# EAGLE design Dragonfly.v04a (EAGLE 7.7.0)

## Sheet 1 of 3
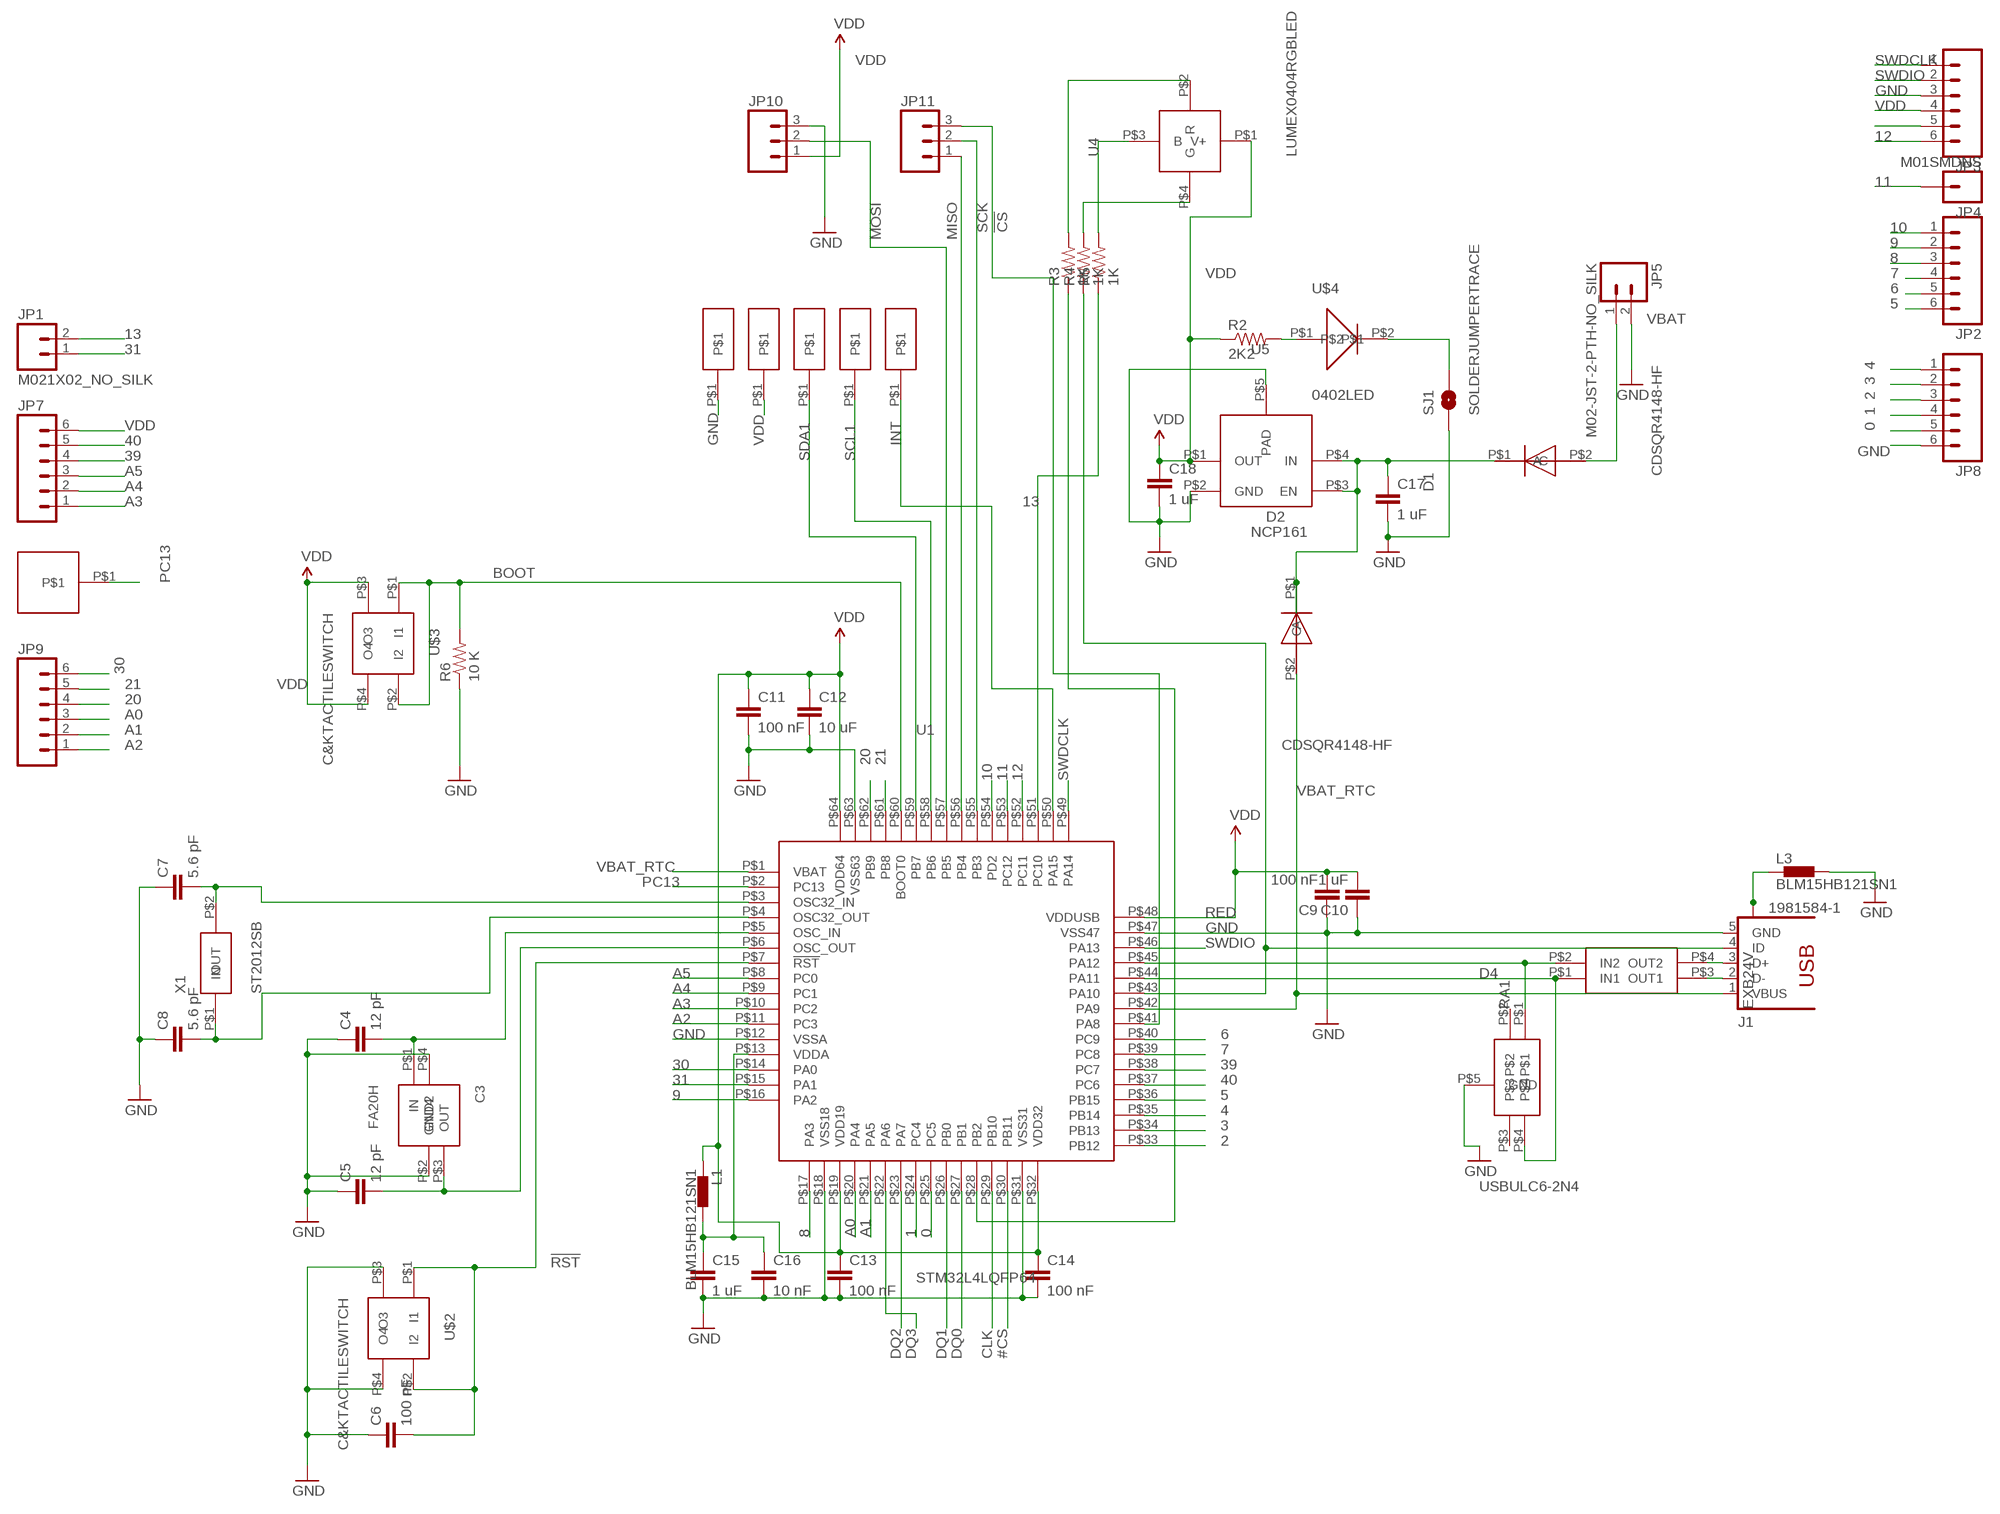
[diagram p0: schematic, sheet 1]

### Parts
C3  FA20H  [FA-20H]
C4  12 pF  0402CAP.KW  [0402-CAP]
C5  12 pF  0402CAP.KW  [0402-CAP]
C6  100 nF  0402CAP.KW  [0402-CAP]
C7  5.6 pF  0402CAP.KW  [0402-CAP]
C8  5.6 pF  0402CAP.KW  [0402-CAP]
C9  100 nF  0402CAP.KW  [0402-CAP]
C10  1 uF  0402CAP.KW  [0402-CAP]
C11  100 nF  0402CAP.KW  [0402-CAP]
C12  10 uF  0402CAP.KW  [0402-CAP]
C13  100 nF  0402CAP.KW  [0402-CAP]
C14  100 nF  0402CAP.KW  [0402-CAP]
C15  1 uF  0402CAP.KW  [0402-CAP]
C16  10 nF  0402CAP.KW  [0402-CAP]
C17  1 uF  0402CAP.KW  [0402-CAP]
C18  1 uF  0402CAP.KW  [0402-CAP]
D1  CDSQR4148-HF  [CDSQR4148-HF]
D2  CDSQR4148-HF  [CDSQR4148-HF]
D4  USBULC6-2N4  [USBULC6-2N4]
J1  1981584-1  [1981584-1]
JP1  M021X02_NO_SILK  [1X02_NO_SILK]
JP2  M06NO_SILK  [1X06_NO_SILK]
JP3  M06NO_SILK  [1X06_NO_SILK]
JP4  M01SMDNS  [1X01NS]
JP5  M02-JST-2-PTH-NO_SILK  [JST-2-PTH-NS]
JP7  M06NO_SILK  [1X06_NO_SILK]
JP8  M06NO_SILK  [1X06_NO_SILK]
JP9  M06NO_SILK  [1X06_NO_SILK]
JP10  M031X03_NO_SILK  [1X03_NO_SILK]
JP11  M031X03_NO_SILK  [1X03_NO_SILK]
L1  BLM15HB121SN1  [0402]
L3  BLM15HB121SN1  [0402]
R2  2K2  0402RES.KW  [0402-RES]
R3  1K  0402RES.KW  [0402-RES]
R4  1K  0402RES.KW  [0402-RES]
R5  1K  0402RES.KW  [0402-RES]
R6  10 K  0402RES.KW  [0402-RES]
RA1  EXB24V  [EXB24V]
SJ1  SOLDERJUMPERTRACE  [SJ_2S-TRACE]
U1  STM32L4LQFP64  [STM32L4LQFP64]
U4  LUMEX0404RGBLED  [LX0404]
U5  NCP161  [NCP161]
U$1  HN01  [HN01]
U$2  C&KTACTILESWITCH  [C&KTACTILESWITCH]
U$3  C&KTACTILESWITCH  [C&KTACTILESWITCH]
U$4  0402LED  [0402LED]
U$5  SMDPAD  [SMDPAD]
U$6  SMDPAD  [SMDPAD]
U$7  SMDPAD  [SMDPAD]
U$8  SMDPAD  [SMDPAD]
U$9  SMDPAD  [SMDPAD]
X1  ST2012SB  [ST2012SB]

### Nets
0: JP8.5 U1.P$25(PC5)
1: JP8.4 U1.P$24(PC4)
2: JP8.3 U1.P$33(PB12)
3: JP8.2 U1.P$34(PB13)
4: JP8.1 U1.P$35(PB14)
5: JP2.6 U1.P$36(PB15)
6: JP2.5 U1.P$40(PC9)
7: JP2.4 U1.P$39(PC8)
8: JP2.3 U1.P$17(PA3)
9: JP2.2 U1.P$16(PA2)
10: JP2.1 U1.P$54(PD2)
11: JP4.1 U1.P$53(PC12)
12: JP3.6 U1.P$52(PC11)
13: JP1.2 R5.1 U1.P$51(PC10)
20: JP9.4 U1.P$62(PB9)
21: JP9.5 U1.P$61(PB8)
30: JP9.6 U1.P$14(PA0)
31: JP1.1 U1.P$15(PA1)
39: JP7.4 U1.P$38(PC7)
40: JP7.5 U1.P$37(PC6)
!CS: JP11.3 U1.P$41(PA8)
!RST: C6.2 U1.P$7(!RST) U$2.P$1(I1) U$2.P$2(I2)
#CS: U1.P$30(PB11) ; also sheet 3
A0: JP9.3 U1.P$20(PA4)
A1: JP9.2 U1.P$21(PA5)
A2: JP9.1 U1.P$11(PC3)
A3: JP7.1 U1.P$10(PC2)
A4: JP7.2 U1.P$9(PC1)
A5: JP7.3 U1.P$8(PC0)
BOOT: R6.2 U1.P$60(BOOT0) U$3.P$1(I1) U$3.P$2(I2)
CLK: U1.P$29(PB10) ; also sheet 3
DQ0: U1.P$27(PB1) ; also sheet 3
DQ1: U1.P$26(PB0) ; also sheet 3
DQ2: U1.P$23(PA7) ; also sheet 3
DQ3: U1.P$22(PA6) ; also sheet 3
GND: C3.P$2(GND2) C3.P$4(GND4) C4.1 C5.1 C6.1 C7.1 C8.1 C9.1 C10.1 C11.2 C12.2 C13.2 C14.2 C15.2 C16.2 C17.2 C18.2 D4.P$5(GND) J1.5(GND) JP3.3 JP5.2 JP8.6 JP10.3 L3.2 R6.1 SJ1.1 U1.P$12(VSSA) U1.P$18(VSS18) U1.P$31(VSS31) U1.P$47(VSS47) U1.P$63(VSS63) U5.P$2(GND) U5.P$5(PAD) U$2.P$3(O3) U$2.P$4(O4) U$7.P$1 ; also sheet 3
INT: U1.P$50(PA15) U$9.P$1
MISO: JP11.1 U1.P$56(PB4)
MOSI: JP10.2 U1.P$57(PB5)
N$1: C7.2 U1.P$3(OSC32_IN) X1.P$2(OUT)
N$2: C8.2 U1.P$4(OSC32_OUT) X1.P$1(IN)
N$3: C3.P$1(IN) C4.2 U1.P$5(OSC_IN)
N$4: C3.P$3(OUT) C5.2 U1.P$6(OSC_OUT)
N$9: C15.1 C16.1 L1.2 U1.P$13(VDDA)
N$11: R3.2 U4.P$2(R)
N$13: SJ1.2 U$4.P$2
N$31: J1.3(D+) RA1.P$4(OUT2)
N$32: J1.4(ID) R4.1 U1.P$43(PA10)
N$33: J1.2(D-) RA1.P$3(OUT1)
N$38: D4.P$1 RA1.P$2(IN2) U1.P$45(PA12)
N$39: D4.P$4 RA1.P$1(IN1) U1.P$44(PA11)
N$42: R2.2 U$4.P$1
N$49: D2.P$2(A) J1.1(VBUS) U1.P$42(PA9)
N$56: R4.2 U4.P$4(G)
N$59: R5.2 U4.P$3(B)
N$60: C17.1 D1.P$1(C) D2.P$1(C) U5.P$3(EN) U5.P$4(IN)
PC13: U1.P$2(PC13) U$1.P$1
RED: R3.1 U1.P$28(PB2)
SCK: JP11.2 U1.P$55(PB3)
SCL1: U1.P$58(PB6) U$6.P$1
SDA1: U1.P$59(PB7) U$5.P$1
SWDCLK: JP3.1 U1.P$49(PA14)
SWDIO: JP3.2 U1.P$46(PA13)
USB_SHIELD: J1.S1 J1.S2 J1.S3 J1.S4 L3.1
VBAT: D1.P$2(A) JP5.1
VBAT_RTC: JP3.5 U1.P$1(VBAT)
VDD: C9.2 C10.2 C11.1 C12.1 C13.1 C14.1 C18.1 JP3.4 JP7.6 JP10.1 L1.1 R2.1 U1.P$19(VDD19) U1.P$32(VDD32) U1.P$48(VDDUSB) U1.P$64(VDD64) U4.P$1(V+) U5.P$1(OUT) U$3.P$3(O3) U$3.P$4(O4) U$8.P$1 ; also sheet 3
Unconnected: D4.P$2 D4.P$3

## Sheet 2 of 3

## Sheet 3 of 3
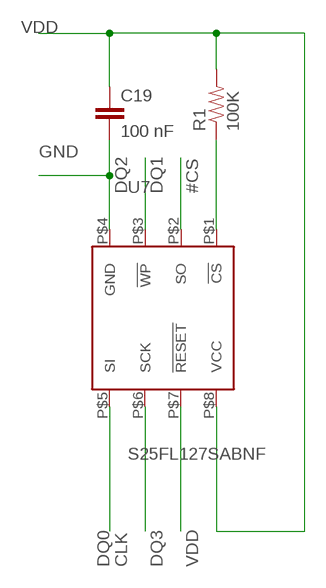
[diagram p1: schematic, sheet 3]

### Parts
C19  100 nF  0402CAP.KW  [0402-CAP]
R1  100K  0402RES.KW  [0402-RES]
U7  S25FL127SABNF  [WSON-8]

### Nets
#CS: R1.1 U7.P$1(!CS) ; also sheet 1
CLK: U7.P$6(SCK) ; also sheet 1
DQ0: U7.P$5(SI) ; also sheet 1
DQ1: U7.P$2(SO) ; also sheet 1
DQ2: U7.P$3(!WP) ; also sheet 1
DQ3: U7.P$7(!RESET) ; also sheet 1
GND: C19.2 U7.P$4(GND) ; also sheet 1
VDD: C19.1 R1.2 U7.P$8(VCC) ; also sheet 1

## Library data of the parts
C3 = Kris:FA20H: Seiko Epson 2.5 mm x 2.0 mm FA-20H 16 MHz crystal
C4-C19 = SparkFun-Capacitors:0402CAP.KW
D1 D2 = Kris:CDSQR4148-HF: ComChip's CDSQR4148-HF high speed 150 mA Io diode
D4 = Kris:USBULC6-2N4: ST TVS diode ESD Protection USBULC6-2N4
J1 = con-usb:1981584-1: Receptacle, micro-USB, type A/B Tyco Electronics; MF: Hirose; MPN: ZX62-AB-5PA(11)
JP1 JP5 = SparkFun-Connectors:M02: Standard 2-pin 0.1" header. Use with
JP2 JP3 JP7-JP9 = SparkFun-Connectors:M06: Header 6 Standard 6-pin 0.1" header. Use with straight break away headers (SKU : PRT-00116), right angle break away headers (PRT-00553), swiss pins (PRT-00743), machine pins (PRT-00117), and female headers (PRT-00115). Molex polarized connector foot print use with SKU : PRT-08094 with associated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
JP4 = SparkFun-Connectors:M01: Header 1
JP10 JP11 = SparkFun-Connectors:M03: Header 3 Standard 3-pin 0.1" header. Use with straight break away headers (SKU : PRT-00116), right angle break away headers (PRT-00553), swiss pins (PRT-00743), machine pins (PRT-00117), and female headers (PRT-00115). Molex polarized connector foot print use with SKU : PRT-08232 with associated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
L1 L3 = inductors:BLM15H: EMIFIL (R) Chip Ferrite Bead for GHz Noise
R1-R6 = SparkFun-Resistors:0402RES.KW
RA1 = Kris:EXB24V: Panasonic EXB24 22 Ohm series resistor pair
SJ1 = SparkFun-Passives:SOLDERJUMPER: Solder Jumper
U1 = Kris:STM32L4LQFP64: LQFP64 Package for ST's STM32L476 32-bit low-power microcontroller
U4 = Kris:LUMEX0404RGBLED: Lumex 0404 rgb leds
U5 = Kris:NCP161: NCP161 3V3 LDO voltage regulator
U7 = Kris:S25FL127SABNF: S225FL127SABNF1101 128 Mbit Spansion flash in WSON-8 package
U$1 = PWSONN6:HN01
U$2 U$3 = Kris:C&KTACTILESWITCH: C&K Tactile Switch 611-PTS810SJS250SMTR
U$4 = Kris:0402LED: 0402led
U$5-U$9 = Kris:SMDPAD: smd test pad
X1 = Kris:ST2012SB: Kyocera 2.0 x 1.2 mm 32.768 20kHz ppm 4 pf crystal

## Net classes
1 USB: width 0.254 mm, drill 0.33 mm, clearance 0.159 mm
2 Top GND Pour: clearance 0.762 mm to class 1

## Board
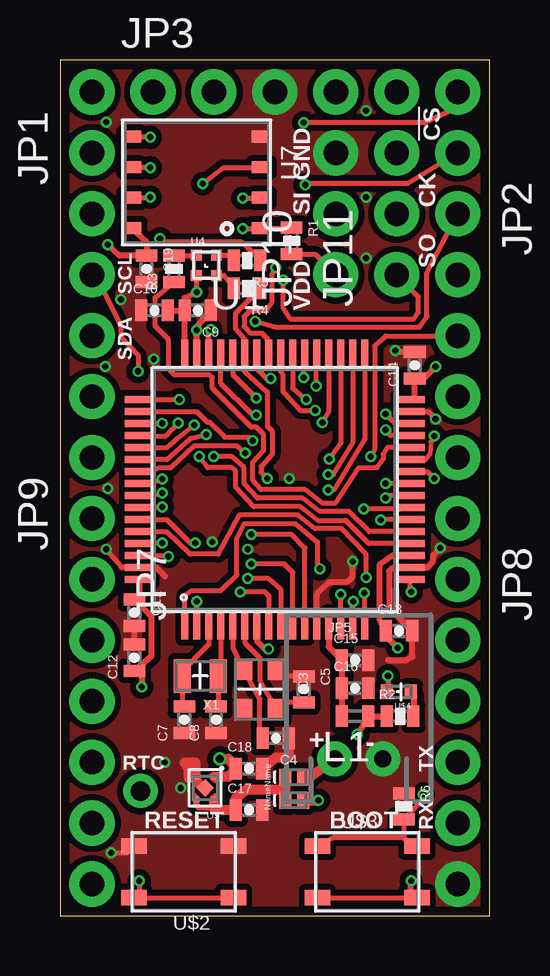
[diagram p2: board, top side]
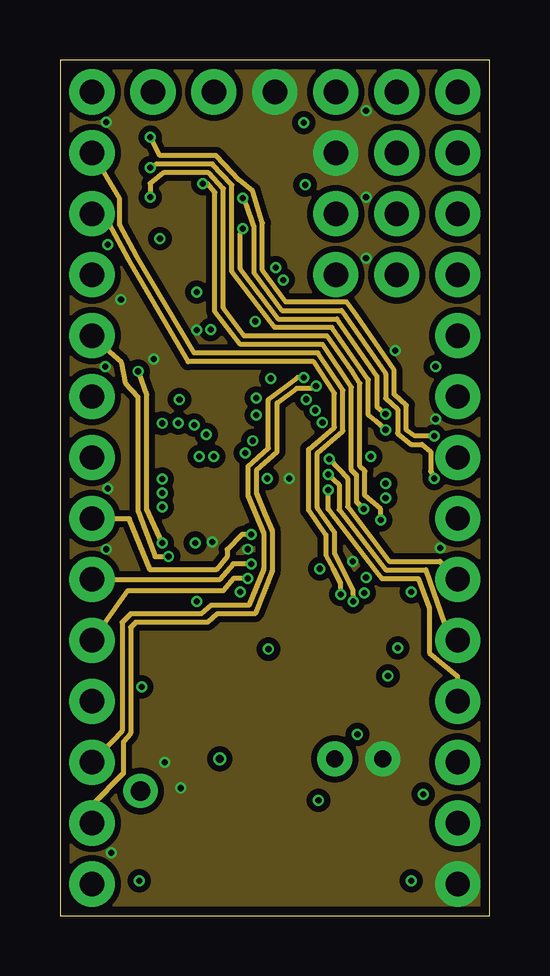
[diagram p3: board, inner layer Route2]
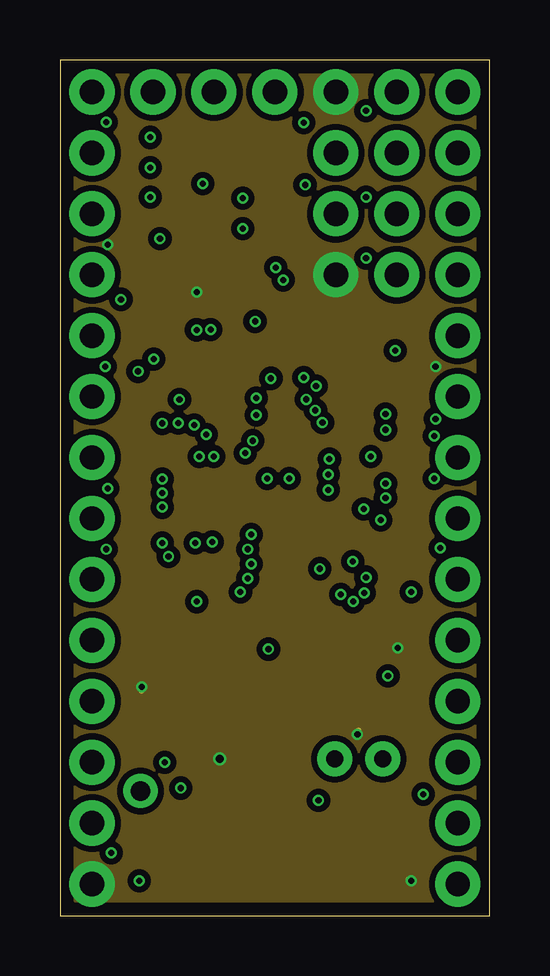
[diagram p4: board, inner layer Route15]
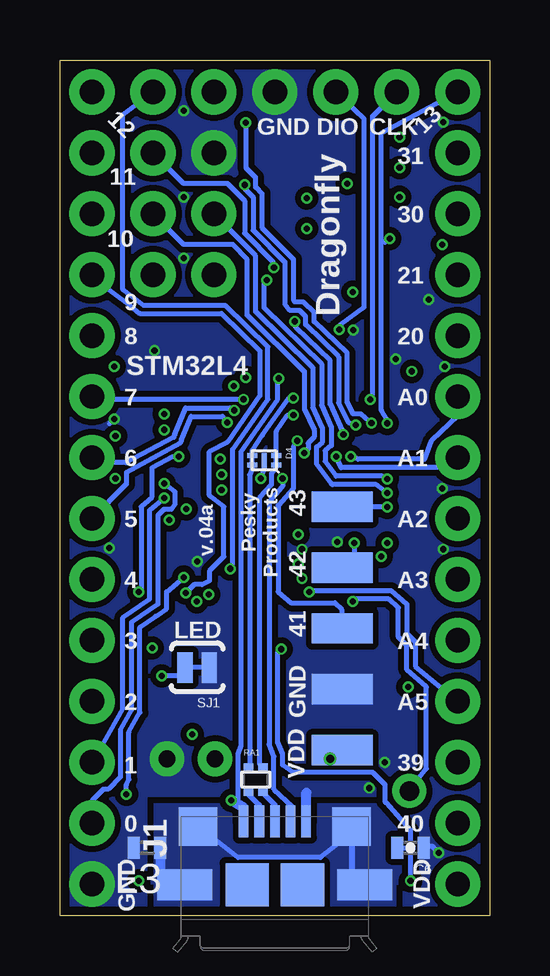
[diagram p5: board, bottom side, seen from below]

Size 17.91 x 35.69 mm. Coordinates in mm from the lower left corner, seen from the top.
Outline: 0,0 17.91,0 17.91,35.69 0,35.69 0,0
Copper layers (1*2*15*16): Top 0.035559375mm / dielectric 0.17018125mm / Route2 0.01778125mm / dielectric 47mil / Route15 0.01778125mm / dielectric 0.17018125mm / Bottom 0.035559375mm
Design rules "OSHPark-4layer *": minimum track width 5mil, minimum drill 10mil, track to track 5mil, track to pad 5mil, pad to pad 5mil, via to via 5mil, smd to smd 5mil, copper to edge 15mil, drill to drill 6mil, minimum pad ring 4mil, minimum via ring 4mil, stop-mask expansion 4mil, vias tented up to drill 20mil, thermal gap 10mil

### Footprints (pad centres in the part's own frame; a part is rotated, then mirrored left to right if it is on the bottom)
FA-20H = smd 0.9 x 0.75: P$1 -0.85,-0.7; P$2 0.85,-0.7; P$3 0.85,0.7; P$4 -0.85,0.7
0402-CAP = smd 0.5 x 0.9: 1 -0.55,0; 2 0.55,0
CDSQR4148-HF = smd 0.7 x 0.5: P$1 0,0.375; P$2 0,-0.375
USBULC6-2N4 = smd 0.2 x 0.4: P$1 0.2,0.5; P$2 -0.2,0.5; P$3 -0.2,-0.5; P$4 0.2,-0.5 | smd 0.6 x 0.2: P$5 0,0
1981584-1 = smd 0.4 x 1.35: 1 -1.3,4.1; 2 -0.65,4.1; 3 0,4.1; 4 0.65,4.1; 5 1.3,4.1 | smd 1.8 x 1.8: M1 -1.15,1.45; M2 1.15,1.45 | smd 2.3 x 1.3: S1 -3.75,1.45; S2 3.75,1.45 | smd 1.6 x 1.6: S3 -3.2,3.885; S4 3.2,3.885
1X02_NO_SILK = drill 1.016 pad 1.88: 1 0,0; 2 2.54,0
1X06_NO_SILK = drill 1.016 pad 1.88: 1 0,0; 2 2.54,0; 3 5.08,0; 4 7.62,0; 5 10.16,0; 6 12.7,0
1X01NS = drill 1.016 pad 1.88: 1 0,0
JST-2-PTH-NS = drill 0.7 pad 1.448: 1 -1,0; 2 1,0
1X03_NO_SILK = drill 1.016 pad 1.88: 1 0,0; 2 2.54,0; 3 5.08,0
0402 = smd 0.5 x 0.9: 1 -0.55,0; 2 0.55,0
0402-RES = smd 0.5 x 0.9: 1 -0.55,0; 2 0.55,0
EXB24V = smd 0.4 x 0.36: P$1 -0.3,0.5; P$2 0.3,0.5; P$3 -0.3,-0.5; P$4 0.3,-0.5
SJ_2S-TRACE = smd 0.635 x 1.27: 1 -0.508,0; 2 0.508,0
STM32L4LQFP64 = smd 0.3 x 1.2: P$1 -3.75,-5.65; P$2 -3.25,-5.65; P$3 -2.75,-5.65; P$4 -2.25,-5.65; P$5 -1.75,-5.65; P$6 -1.25,-5.65; P$7 -0.75,-5.65; P$8 -0.25,-5.65; P$9 0.25,-5.65; P$10 0.75,-5.65; P$11 1.25,-5.65; P$12 1.75,-5.65; P$13 2.25,-5.65; P$14 2.75,-5.65; P$15 3.25,-5.65; P$16 3.75,-5.65; P$33 3.75,5.65; P$34 3.25,5.65; P$35 2.75,5.65; P$36 2.25,5.65; P$37 1.75,5.65; P$38 1.25,5.65; P$39 0.75,5.65; P$40 0.25,5.65; P$41 -0.25,5.65; P$42 -0.75,5.65; P$43 -1.25,5.65; P$44 -1.75,5.65; P$45 -2.25,5.65; P$46 -2.75,5.65; P$47 -3.25,5.65; P$48 -3.75,5.65 | smd 1.2 x 0.3: P$17 5.65,-3.75; P$18 5.65,-3.25; P$19 5.65,-2.75; P$20 5.65,-2.25; P$21 5.65,-1.75; P$22 5.65,-1.25; P$23 5.65,-0.75; P$24 5.65,-0.25; P$25 5.65,0.25; P$26 5.65,0.75; P$27 5.65,1.25; P$28 5.65,1.75; P$29 5.65,2.25; P$30 5.65,2.75; P$31 5.65,3.25; P$32 5.65,3.75; P$49 -5.65,3.75; P$50 -5.65,3.25; P$51 -5.65,2.75; P$52 -5.65,2.25; P$53 -5.65,1.75; P$54 -5.65,1.25; P$55 -5.65,0.75; P$56 -5.65,0.25; P$57 -5.65,-0.25; P$58 -5.65,-0.75; P$59 -5.65,-1.25; P$60 -5.65,-1.75; P$61 -5.65,-2.25; P$62 -5.65,-2.75; P$63 -5.65,-3.25; P$64 -5.65,-3.75
LX0404 = smd 0.45 x 0.45: P$1 -0.425,-0.425; P$2 -0.425,0.425; P$3 0.425,0.425; P$4 0.425,-0.425
NCP161 = smd 0.24 x 0.24: P$1 -0.37,-0.48; P$2 0.37,-0.48; P$3 0.37,0.48; P$4 -0.37,0.48 | smd 0.52 x 0.52 rotated 45: P$5 0,0
WSON-8 = smd 0.5 x 0.8: P$1 1.905,2.7; P$2 0.635,2.7; P$3 -0.635,2.7; P$4 -1.905,2.7; P$5 -1.905,-2.7; P$6 -0.635,-2.7; P$7 0.635,-2.7; P$8 1.905,-2.7
HN01 = drill 0.813 pad 1.422: P$1 0,0
C&KTACTILESWITCH = smd 1.05 x 0.65: P$1 -2.075,1.073; P$2 2.075,1.075; P$3 -2.075,-1.075; P$4 2.075,-1.075
0402LED = smd 0.5 x 0.6: P$1 -0.5,0; P$2 0.5,0
SMDPAD = smd 1.27 x 2.54: P$1 0,0
ST2012SB = smd 0.7 x 1.4: P$1 -0.75,0; P$2 0.75,0

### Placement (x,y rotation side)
C3  8.33,9.45 270 top
C4  8.99,7.42 180 top
C5  10.16,9.45 270 top
C6  3.3,2.84 180 bottom
C7  5.18,8.18 90 top
C8  6.5,8.18 90 top
C9  5.74,25.25 180 top
C10  3.94,25.25 0 top
C11  3.1,12.65 270 top
C12  3.1,10.77 90 top
C13  14.12,11.89 0 top
C14  14.78,22.96 90 top
C15  12.29,10.67 0 top
C16  12.29,9.5 0 top
C17  7.87,4.42 0 top
C18  7.87,6.15 0 top
C19  3.61,26.97 270 top
D1  9.75,5.79 90 top
D2  9.75,4.83 90 top
D4  9.4,19 270 bottom
J1  8.95,-0.15 0 bottom
JP1  1.33,31.81 90 top
JP2  16.57,29.27 270 top
JP3  3.87,34.35 0 top
JP4  16.57,31.81 0 top
JP5  12.45,6.55 0 top
JP7  1.33,14.03 270 top
JP8  16.57,14.03 270 top
JP9  1.33,16.57 90 top
JP10  11.49,26.73 90 top
JP11  14.03,26.73 90 top
L1  12.29,8.33 180 top
L3  14.27,2.84 180 bottom
R1  9.65,28.14 270 top
R2  14.17,8.33 0 top
R3  4.75,26.97 90 top
R4  7.8,26.16 180 top
R5  7.8,27.33 180 top
R6  14.33,4.57 270 top
RA1  9.75,5.69 0 bottom
SJ1  12.19,10.36 180 bottom
U1  8.95,17.78 0 top
U4  6.1,27.13 0 top
U5  6.05,5.33 180 top
U7  5.69,30.58 270 top
U$1  3.35,5.21 0 top
U$2  5.16,1.84 180 top
U$3  12.8,1.84 0 top
U$4  14.12,9.35 180 top
U$5  6.15,14.53 270 bottom
U$6  6.15,17.07 270 bottom
U$7  6.15,9.45 270 bottom
U$8  6.15,6.91 270 bottom
U$9  6.15,11.99 270 bottom
X1  5.84,10.01 180 top

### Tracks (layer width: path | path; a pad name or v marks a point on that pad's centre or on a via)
0  (via drill 0.25)
  Top 0.203: U1.P$25 13.62,18.03 v13.56,18.03
  Bottom 0.203: v13.56,18.03 13.11,17.68 13.11,17.17 13.26,16.97 13.56,16.97 13.82,16.71 13.82,13.01 14.94,12.24 14.94,8.59 15.39,7.77 15.39,5.79 15.9,5.28 16.1,5.28 16.56,4.83 16.56,3.89 JP8.5
1  (via drill 0.25)
  Top 0.203: U1.P$24 13.77,17.53 v13.56,17.42
  Bottom 0.203: v13.56,17.42 14.17,16.92 14.17,13.21 15.29,12.45 15.29,8.66 JP8.4
2  (via drill 0.25)
  Top 0.203: U1.P$33 12.7,19.87 11.42,17.77 v11.18,17.77
  Route2 0.203: v11.18,17.77 11.18,16.97 13.16,14.38 13.41,14.07 14.94,14.07 15.39,12.85 15.39,10.97 16.56,10.01 16.56,8.97 JP8.3
3  (via drill 0.25)
  Top 0.203: U1.P$34 12.2,20.18 12.19,19.71 11.39,18.4 v11.18,18.4
  Route2 0.203: v11.18,18.4 11.63,17.98 11.63,16.94 13.56,14.43 15.24,14.43 16.18,11.73 16.33,11.73 JP8.2
4  (via drill 0.25)
  Top 0.203: U1.P$35 11.7,19.72 v11.23,19.05
  Route2 0.203: v11.23,19.05 11.99,18.24 11.99,17.07 13.72,14.78 15.82,14.78 JP8.1
5  (via drill 0.25)
  Top 0.203: U1.P$36 11.2,21.03 v10.94,20.57
  Bottom 0.203: v10.94,20.57 11.14,20.83 12.45,20.83 12.85,19.81 12.9,19.71 15.14,18.49 15.14,18.01 JP2.6
6  (via drill 0.25)
  Top 0.203: v10.64,21.08 10.01,21.08 9.29,21.85 9.29,22.56 9.2,22.71 U1.P$40
  Bottom 0.203: v10.64,21.08 10.82,21.18 12.68,21.18 13.12,20.07 13.16,19.96 15.16,18.9 16.38,18.9 16.57,19.09 JP2.5
7  (via drill 0.25)
  Top 0.203: U1.P$39 9.69,22.01 10.01,21.74 v10.26,21.54
  Bottom 0.203: v10.26,21.54 16.46,21.54 JP2.4
8  (via drill 0.25)
  Top 0.203: v14.63,13.51 14.59,13.57 14.59,14.02 U1.P$17 | JP2.3 16.43,24.18 13.56,24.18 13.11,23.77 13.11,19.46 v12.95,19.15
  Bottom 0.203: v12.95,19.15 13.21,19.15 14.07,18.69 14.07,17.48 14.53,17.07 14.53,13.56 v14.63,13.51
9  (via drill 0.25)
  Top 0.203: U1.P$16 12.69,13.32 v12.68,13.46
  Bottom 0.203: v12.68,13.46 12.32,13.82 11.99,13.82 11.68,13.97 11.68,14.38 11.07,14.99 11.07,17.07 11.68,17.53 11.68,19.36 10.92,19.76 9.58,21.69 9.58,23.57 11.18,25.12 14.58,25.12 14.99,25.45 15.8,26.06 16.57,26.63 JP2.2
10  (via drill 0.25)
  Top 0.203: v6.1,20.07 5.44,19.91 4.45,19.03 U1.P$54 | v8.13,24.79 8.99,24.54 14.96,24.54 15.29,24.99 15.29,26.82 JP2.1
  Bottom 0.203: v8.13,24.79 8.08,24.54 6.66,23.16 6.66,21.34 6.15,20.22 v6.1,20.07
11  (via drill 0.25)
  Top 0.203: U1.P$53 4.44,19.53 4.88,19.91 v5.59,20.47 | v10.21,30.48 10.31,30.53 14.48,30.53 JP4.1
  Bottom 0.203: v10.21,30.48 10.21,30.33 9.86,29.97 9.86,28.59 8.53,27.27 8.53,25.5 8.33,25.25 7.92,25.25 7.67,24.99 7.67,24.65 6.3,23.32 6.3,21.39 5.89,20.57 v5.59,20.47
12  (via drill 0.25)
  Top 0.203: JP3.6 16.57,33.69 15.19,33.07 v10.16,33.07 | 3.23,20.02 3.3,20.02 | 3.3,20.02 4.42,20.02 v4.93,20.55 | U1.P$52 3.3,20.02
  Bottom 0.203: v4.93,20.55 5.18,20.75 5.38,20.93 5.69,20.93 5.94,21.44 5.94,23.47 7.32,24.78 7.32,25.15 7.77,25.6 8.13,25.6 8.18,25.7 8.18,27.38 9.5,28.7 9.5,30.12 9.75,30.38 9.75,30.79 10.16,31.19 v10.16,33.07
13  (via drill 0.25)
  Top 0.203: 4.11,20.53 v4.27,20.54 | U1.P$51 4.16,20.53 | v4.17,28.25 4.37,28.09 7.57,28.09 7.8,27.89 8,27.68 R5.1
  Top 0.254: 4.16,20.53 v4.27,20.54
  Bottom 0.203: v4.27,20.54 4.22,20.62 4.27,20.68 4.52,21.08 4.52,28.09 | 4.52,28.09 4.52,32.64 JP1.2 | v4.17,28.25 4.37,28.09 4.52,28.09
20  (via drill 0.25)
  Top 0.203: U1.P$62 4.36,15.03 v4.52,14.99
  Route2 0.203: v4.52,14.99 3.96,14.99 3.25,16.87 3.25,21.64 2.74,22.2 2.56,23.06 1.6,23.93 JP9.4
21  (via drill 0.25)
  Top 0.203: v4.27,15.54 4.2,15.53 U1.P$61 | JP9.5 1.46,26.73 2.54,24.64 2.54,24.13 3.25,23.37 v3.25,22.71
  Route2 0.203: v4.27,15.54 3.61,16.97 3.61,21.69 v3.25,22.71
30  (via drill 0.25)
  Top 0.203: U1.P$14 v11.7,13.4
  Route2 0.203: JP9.6 2.03,28.88 2.85,27.38 5.33,23.11 10.57,23.11 11.43,21.79 11.43,20.37 10.36,19.46 10.36,16.92 11.08,15.89 11.08,15.04 11.38,14.48 11.68,13.87 v11.7,13.4
31  (via drill 0.25)
  Top 0.254: U1.P$15 12.19,12.96 v12.21,13.11
  Route2 0.203: v12.21,13.11 12.19,13.61 11.43,15.14 11.43,16 10.72,17.02 10.72,19.3 11.79,20.22 11.79,21.92 10.74,23.47 5.59,23.47 3.2,27.48 2.49,28.8 2.49,29.9 JP1.1
39  (via drill 0.25)
  Top 0.203: v10.16,22.45 10.16,23.4 U1.P$38
  Route2 0.152: 1.37,6.45 JP7.4
  Route2 0.203: v10.16,22.45 9.91,22.45 8.69,21.54 8.69,19.51 7.82,18.75 7.82,17.53 8.48,15.95 8.48,14.48 7.87,12.95 6.3,12.95 5.89,12.6 2.95,12.6 2.59,12.24 2.59,7.72 JP7.4
40  (via drill 0.25)
  Top 0.203: v10.67,22.1 10.67,23.4 U1.P$37
  Route2 0.203: v10.67,22.1 10.46,22 9.86,22 9.04,21.39 9.04,19.36 8.18,18.59 8.18,17.63 8.53,16.76 8.84,16.05 8.84,14.38 8.13,12.6 6.55,12.6 6.15,12.24 3.15,12.24 2.95,12.04 2.95,7.62 2.64,7.26 2.64,5.94 1.32,4.62 1.32,3.89 JP7.5
!CS  (via drill 0.25)
  Top 0.203: U1.P$41 8.64,24.07 8.43,24.28 7.98,24.28 7.67,24.59 7.67,24.99 7.92,25.25 8.59,25.25 8.84,25.6 8.84,26.77 v8.99,27.03
  Bottom 0.203: JP11.3 12.75,30.53 10.92,30.53 10.21,29.82 10.21,28.46 9.04,27.28 v8.99,27.03
!RST  (via drill 0.25)
  Top 0.203: 3.3,0.77 6.92,0.77 | v3.3,1.47 3.3,0.77 | 3.3,0.77 U$2.P$2
  Top 0.254: U1.P$7 8.2,11.47 8.53,11.12 v8.69,11.12 | 6.92,0.77 U$2.P$1
  Bottom 0.203: v3.3,1.47 3.3,2.85 | 3.3,2.85 3.3,3.56 4.32,4.72 4.37,4.78 4.37,5.49 4.88,5.99 8.18,5.99 8.64,6.3 8.64,6.76 8.84,7.26 8.84,10.97 v8.69,11.12 | C6.2 3.3,2.85
#CS  (via drill 0.25)
  Top 0.203: U1.P$30 13.96,20.53 v13.56,20.93 | v7.62,28.65 8.16,28.65 U7.P$1 9.69,28.68 R1.1
  Route2 0.203: v13.56,20.93 13.21,21.23 13.21,22.5 11.63,24.74 11.53,24.89 9.09,24.89 7.52,26.98 7.52,28.45 v7.62,28.65
A0  (via drill 0.25)
  Top 0.203: U1.P$20 12.87,15.53 11.9,16.5 10.73,16.5 10.01,17.07 8.08,17.07 7.32,17.88 7.32,18.54 7.16,18.69 6.15,18.69 v5.8,19.15
  Bottom 0.203: v5.8,19.15 5.49,19.05 2.72,19.05 2.41,19.84 1.32,20.88 JP9.3
A1  (via drill 0.25)
  Top 0.203: U1.P$21 12.88,16.03 12.04,16.87 10.82,16.87 10.11,17.42 8.23,17.42 7.67,18.03 7.67,18.69 7.16,19.15 v6.4,19.15
  Bottom 0.203: v6.4,19.15 6.2,18.69 1.75,18.69 JP9.2
A2  (via drill 0.25)
  Top 0.203: U1.P$11 10.2,15.35 9.65,15.9 v7.98,15.9
  Route2 0.203: v7.98,15.9 7.57,15.9 6.96,15.29 6.96,14.99 6.5,14.43 3.76,14.43 2.9,16.56 1.35,16.56 JP9.1
A3  (via drill 0.25)
  Top 0.203: U1.P$10 9.7,14.32 9.35,14.68 v7.98,14.68
  Route2 0.203: JP7.1 1.73,14.02 6.66,14.02 7.21,14.68 v7.98,14.68
A4  (via drill 0.25)
  Top 0.203: U1.P$9 9.2,13.61 8.69,14.07 v7.82,14.07
  Route2 0.203: JP7.2 2.5,13.13 2.83,13.56 6.81,13.56 7.21,14.07 v7.82,14.07
A5  (via drill 0.25)
  Top 0.203: U1.P$8 8.7,13.34 8.53,13.51 v7.52,13.51
  Bottom 0.203: v7.52,13.51 7.32,13.56 4.12,13.56 3.45,13.01 3.45,11.79 3.1,11.43 3.1,10.41 JP7.3
BOOT  (via drill 0.25)
  Top 0.203: U1.P$60 4.44,16.03 5.44,15.09 6.6,15.09 7.47,16.71 9.91,16.71 10.62,16.15 11.73,16.15 12.75,15.09 v12.75,14.12 | 14.61,2.92 14.66,2.92 14.33,3.25 | 14.33,3.25 11.37,3.25 U$3.P$1 | U$3.P$2 14.88,3.14 15.24,3.15 | 14.33,3.25 R6.2 15.13,4.88 v15.14,5.08
  Top 0.254: U$3.P$2 14.61,2.92 | 11.07,3.1 10.91,3.1 U$3.P$1
  Bottom 0.203: v12.75,14.12 13.46,13.51 13.46,12.8 13.82,12.55 13.92,12.5 14.58,12.04 14.58,8.48 15.04,7.67 15.04,5.69 15.14,5.49 v15.14,5.08
CLK  (via drill 0.25)
  Top 0.203: U1.P$29 13.78,20.03 v13.56,20.27 | U7.P$6 3.79,31.22 v3.76,31.19
  Route2 0.203: v13.56,20.27 13.16,20.62 12.85,20.88 12.85,22.35 11.33,24.54 8.94,24.54 8.23,25.45 7.16,26.87 7.16,30.48 6.35,31.34 4.01,31.34 v3.76,31.19
DQ0  (via drill 0.25)
  Top 0.178: 15.22,19.03 15.42,19.25 15.47,19.76
  Top 0.203: 15.47,19.76 v15.6,20.02 | U1.P$27 15.22,19.03 | U7.P$5 3.79,32.49 v3.76,32.46
  Route2 0.203: v15.6,20.02 14.78,20.02 14.43,20.27 14.43,21.29 13.92,21.74 13.92,22.76 12.34,25.04 11.94,25.6 9.4,25.6 8.43,26.92 8.43,28.91 8.03,30.23 7.47,30.68 6.5,31.7 4.17,31.7 v3.76,32.46
DQ1  (via drill 0.25)
  Top 0.203: U1.P$26 15.3,18.53 v15.6,18.24 | v7.62,29.92 8.36,29.92 U7.P$2
  Route2 0.203: v15.6,18.24 15.44,18.54 15.44,19.36 15.09,19.66 14.63,19.66 14.07,20.12 14.07,21.13 13.56,21.59 13.56,22.61 11.73,25.25 9.25,25.25 8.08,26.82 8.08,28.75 7.77,29.62 v7.62,29.92
DQ2  (via drill 0.25)
  Top 0.203: U1.P$23 14.24,17.03 14.17,16.97 v12.65,16.97 | v5.94,30.53 6.81,31.19 8.36,31.19 U7.P$3
  Route2 0.203: v12.65,16.97 12.34,17.27 12.34,18.39 12.14,18.59 12.14,22.05 10.95,23.82 7.52,23.82 6.45,25.2 6.45,30.18 6.15,30.53 v5.94,30.53
DQ3  (via drill 0.25)
  Top 0.203: U1.P$22 13.44,16.53 v13.36,16.51 | U7.P$7 3.79,29.95 v3.76,29.97
  Route2 0.203: v13.36,16.51 13.36,16.97 12.7,17.53 12.7,18.54 12.5,18.75 12.5,22.2 12.14,22.76 11.12,24.18 7.67,24.18 6.81,25.35 6.81,30.33 6.2,30.99 4.32,30.99 3.76,30.53 v3.76,29.97
GND  (via drill 0.25)
  Top 0.203: U1.P$31 15.34,21.03 v15.65,20.73 | C5.1 9.43,10 C3.P$4 | U1.P$63 2.59,14.53 v1.93,15.29 | 3.11,11.96 C11.2 | 3.39,26.29 C19.2 | v9.55,18.24 9.55,18.14 | v2.13,2.64 2.81,2.64 U$2.P$4
  Top 0.254: 5.69,24.13 5.64,24.5 C9.1 | U1.P$47 5.69,24.13 | 5.69,24.13 v5.69,24.43 | U1.P$63 4.01,14.53 4.37,14.17 | C14.2 13.91,23.51 v13.97,23.57 | U$2.P$3 7.23,3.12 | 13.66,10.67 14.43,10.67 14.68,10.82 14.68,11.83 C13.2 13.72,12.84 13.72,14.38 13.87,14.53 U1.P$18 15.29,14.53 15.54,14.78 15.54,15.04 v15.85,15.34 | C12.2 3.11,11.96 | U1.P$12 10.7,13.33 10.7,13.43 11.23,13.92 11.94,13.92 12.19,14.12 v12.19,14.78
  Top 0.406: C18.2 8.43,6.15 8.99,6.6 9.45,6.6 9.55,6.66 9.55,7.41 C4.1 | U5.P$2 5.37,6.16 | 5.37,5.75 5.37,6.16 | 5.37,6.16 5.18,6.4 5.64,6.4 5.64,5.69 5.89,5.44 5.94,5.44 U5.P$5
  Bottom 0.203: v15.65,20.73 15.85,20.52 | D4.P$5 9.4,18.69 v9.55,18.24 | C6.1 2.71,2.85 2.62,2.92 2.41,2.92 v2.13,2.64
  Bottom 0.254: v13.97,23.57 13.87,23.52
  Bottom 0.406: J1.5 7.64,5.15
  other vias: 6.35,15.6 1.93,33.1 1.98,17.83 1.88,22.91 7.82,15.29 12.75,27.43 12.75,29.97 4.37,6.4 12.75,33.58 2.54,25.7 3.91,23.22 5.03,5.33
  pour Route2 (isolate 0.254, no thermals): 0,35.69 17.91,35.69 17.91,0 0,0
  pour Bottom (isolate 0.254, no thermals): 3.56,0 0,0 0,35.69 17.91,35.69 17.91,0 14.33,0 14.33,5.03 3.56,5.03
  pour Top (isolate 0.254, no thermals): 0,35.69 17.91,35.69 17.91,0 0,0
INT  (via drill 0.25)
  Top 0.203: U1.P$50 5.69,21.03 6.15,20.57 6.25,20.57 6.86,19.96 7.87,19.96 v8.03,19.81
  Bottom 0.203: v8.03,19.81 8.18,19.56 8.18,17.83 8.81,17.12 8.81,13.51 8.28,13.06 6.45,13.06 6.15,12.75 U$9.P$1
MISO  (via drill 0.25)
  Top 0.203: U1.P$56 3.75,18.03 v4.27,18.21 | v9.3,26.52 9.3,25.35 9.6,24.89 14.73,24.89 14.94,25.17 14.94,25.83 JP11.1
  Bottom 0.203: v4.27,18.21 4.47,18.34 6.4,18.34 6.86,18.95 6.86,19.41 6.6,19.61 6.6,20.37 7.01,21.29 7.01,23.01 9.4,25.35 9.4,26.42 v9.3,26.52
MOSI  (via drill 0.25)
  Top 0.203: U1.P$57 3.81,17.53 v4.27,17.63
  Bottom 0.203: v4.27,17.63 4.72,17.98 6.55,17.98 6.6,18.03 7.21,18.85 7.21,19.56 6.96,19.76 6.96,20.32 7.37,21.23 7.37,22.86 7.42,22.91 9.75,25.2 9.75,27.52 JP10.2
N$1
  Top 0.203: U1.P$3 6.2,11.31 4.99,10.1 X1.P$2 5.09,8.82 C7.2
N$2
  Top 0.203: U1.P$4 6.7,10.12 X1.P$1 6.59,8.77 C8.2
N$3
  Top 0.203: U1.P$5 7.2,11.2 C3.P$1 8.33,9.04 8.33,7.82 8.34,7.68 C4.2
N$4
  Top 0.203: U1.P$6 7.7,11.38 8.02,11.08 8.33,10.77 8.33,9.81 C3.P$3 9.18,8.9 C5.2
N$9
  Top 0.254: L1.2 C16.1 C15.1 11.19,11.22 U1.P$13
N$11
  Top 0.203: R3.2 5.44,27.52 U4.P$2
N$13  (via drill 0.25)
  Top 0.203: v13.66,10.01 13.67,9.7 U$4.P$2
  Bottom 0.203: SJ1.2 12.85,10.01 v13.66,10.01
N$31
  Bottom 0.203: J1.3 8.95,4.64 9.45,5.14 RA1.P$4
N$32  (via drill 0.25)
  Top 0.203: v8.64,18.24 8.38,18.49 8.38,18.75 8.84,19.25 8.84,20.22 8.64,20.42 8.64,21.84 7.69,22.69 U1.P$43 7.7,24.05 7.32,24.49 7.32,25.13 R4.1
  Bottom 0.203: J1.4 8.24,4.01 8.23,4.02 8.23,4.57 8.99,5.28 8.99,6.66 9.2,7.16 9.2,17.27 8.66,17.88 8.64,17.91 v8.64,18.24
N$33
  Bottom 0.203: J1.2 9.6,4.64 9.62,4.64 10.06,5.08 RA1.P$3
N$38  (via drill 0.25)
  Top 0.203: v8.18,20.88 8.03,20.88 6.71,22.2 U1.P$45
  Bottom 0.203: RA1.P$2 9.58,6.32 9.58,17.45 9.09,17.98 9.09,18.45 8.9,18.7 D4.P$1 8.9,20.21 8.43,20.88 v8.18,20.88
N$39  (via drill 0.25)
  Top 0.203: v8.18,21.59 7.21,22.55 7.21,23.42 U1.P$44
  Bottom 0.203: 9.98,6.26 10.01,6.24 | v8.18,21.59 8.38,21.59 9.47,20.04 9.9,19.41 D4.P$4 9.9,18.65 10.01,18.39 10.01,6.24 | 10.01,6.24 RA1.P$1
N$42
  Top 0.254: R2.2 14.77,9.2 U$4.P$1
N$49  (via drill 0.25)
  Top 0.203: U1.P$42 8.19,22.82 8.62,22.41 v8.79,22.41
  Top 0.406: D2.P$2 v10.77,4.83
  Bottom 0.203: v8.79,22.41 8.84,22.35 8.84,21.54 10.36,19.36 10.36,7.11 10.49,6.76 10.49,4.67 10.26,4.5 J1.1
  Bottom 0.406: J1.1 10.25,4.51 v10.77,4.83
N$56
  Top 0.203: U4.P$4 6.83,26.7 R4.2
N$59
  Top 0.203: U4.P$3 7.31,27.55 R5.2
N$60
  Top 0.254: U5.P$3 5.67,4.64 5.79,4.52 6.4,4.52
  Top 0.406: U5.P$4 6.42,4.54 6.4,4.52 6.76,4.42 C17.1 7.32,4.94 7.77,5.28 9.38,5.28 | D1.P$1 9.38,5.28 | 9.38,5.28 D2.P$1
PC13  (via drill 0.25)
  Top 0.203: U1.P$2 v5.7,13.11
  Bottom 0.203: v5.7,13.11 5.59,13.21 4.22,13.21 3.81,12.85 3.81,11.63 3.45,11.28 3.45,10.26 2.64,9.55 2.64,6.15 3.28,5.32 3.33,5.28 U$1.P$1
RED
  Top 0.203: R3.1 3.96,25.79 3.96,24.59 4.52,24.03 4.52,22.81 4.78,22.55 6.21,22.55 6.35,22.47 6.35,22.01 7.98,20.38 8.18,20.38 8.48,20.07 8.48,19.41 8.03,18.9 8.03,18.19 8.38,17.78 10.21,17.78 10.92,17.22 11.48,17.22 12.45,18.69 13.21,18.69 13.46,19.05 13.46,19.25 13.64,19.53 U1.P$28
SCK  (via drill 0.25)
  Top 0.203: U1.P$55 3.85,18.53 4.12,18.69 4.62,18.69 5.6,19.61 7.37,19.61 v7.72,19.3
  Bottom 0.203: JP11.2 12.75,27.99 10.69,27.99 10.11,27.38 10.11,25.04 7.72,22.71 7.72,21.13 7.32,20.27 7.32,19.96 7.57,19.71 7.57,19.46 v7.72,19.3
SCL1  (via drill 0.25)
  Top 0.203: U1.P$58 v4.27,17.04
  Bottom 0.203: v4.27,17.04 6.12,17.04 U$6.P$1
SDA1  (via drill 0.25)
  Top 0.203: U1.P$59 4.45,16.53 5.44,15.54 v5.64,15.54
  Bottom 0.203: v5.64,15.54 5.64,15.04 U$5.P$1
SWDCLK  (via drill 0.25)
  Top 0.203: U1.P$49 4.89,21.53 v4.98,21.53
  Bottom 0.203: v4.98,21.53 4.88,21.74 4.88,33.35 JP3.1
SWDIO  (via drill 0.25)
  Top 0.203: U1.P$46 6.2,24.37 v6.27,24.44
  Bottom 0.203: JP3.2 5.23,33.22 5.23,25.38 6.25,24.64 6.25,24.47 v6.27,24.44
USB_SHIELD
  Bottom 0.203: 5.69,3.5 7.06,2.44 10.49,2.44 J1.S3
  Bottom 0.254: J1.S4 5.75,1.85 J1.S2
  Bottom 0.406: L3.1 13.72,1.84 13.31,1.42 12.77,1.42 J1.S1 | J1.S4 5.69,3.5
  pour Bottom (isolate 0.254, rank 3, no thermals): 14.3,0 14.3,4.98 3.53,4.98 3.53,0
VBAT
  Top 0.406: 11.43,6.54 JP5.1 10.43,5.79 D1.P$2
VBAT_RTC  (via drill 0.25)
  Top 0.203: U1.P$1 5.2,13.36 5.49,13.56 6.71,13.56 7.37,14.22 7.37,15.75 7.67,16.36 9.8,16.36 10.72,15.6 10.72,14.68 v10.82,14.48
  Bottom 0.203: JP3.5 15.29,33.4 15.29,26.11 14.43,25.45 11.02,25.45 9.25,23.72 9.25,21.54 10.72,19.46 10.72,14.68 v10.82,14.48
VDD  (via drill 0.25, 0.33)
  Top 0.203: 13.31,12.35 13.56,11.79 13.57,11.78 | U$3.P$3 U$3.P$4 | U4.P$1 5.67,26.09 v5.7,26.01 | U7.P$8 2.99,28.66 | R1.2 10.63,27.59 JP10.1
  Top 0.254: U1.P$64 3.3,13.39 C11.1 3.16,13.2 3.81,12.5 3.81,10.83 C12.1 3.4,10.02 v3.4,9.55 | U$3.P$4 14.62,1.06 v14.63,1.47 | U1.P$48 5.19,24.94 C9.2 | C9.2 5.19,25.76 v5.7,26.01 | C10.2 C9.2 | U1.P$19 13.86,15.03 13.31,14.63 13.31,12.35 C13.1 | v15.65,22.91 15.15,22.41 C14.1 14.78,21.61 U1.P$32 | 13.57,11.78 13.57,11.68 v14.07,11.18 | 13.72,8.34 R2.1 L1.1 12.79,8.22 v12.39,7.57 | 2.99,28.66 3.61,28.09 C19.1 2.5,27.52 v1.98,27.99
  Top 0.406: U5.P$1 7.04,5.81 C18.1 7.02,6.55 v6.66,6.55
  Route15 0.254: v14.63,1.47 14.53,1.52 | v5.7,26.01 5.79,26.01 | v15.65,22.91 15.7,22.96 | v14.07,11.18 14.12,11.12 14.17,11.23 | v12.39,7.57 12.45,7.72 | v1.98,27.99 1.93,28.04 | v3.4,9.55 3.4,9.4
  Bottom 0.203: v6.66,6.55 6.2,6.55 U$8.P$1
  pour Route15 (isolate 0.254, no thermals): 0.64,35.05 17.27,35.05 17.27,0.64 0.64,0.64

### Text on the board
tPlace: !CS | GND | CK | SI | SCL | SO | VDD | SDA | - | + | TX | RTC | RX | RESET | BOOT
bPlace: 13 | CLK | DIO | GND | 12 | 31 | 11 | 30 | 10 | 21 | Dragonfly | 9 | 20 | 8 | STM32L4 | A0 | 7 | A1 | 6 | 43 | Pesky / Products | v.04a | A2 | 5 | 42 | A3 | 4 | 41 | LED | A4 | 3 | GND | A5 | 2 | VDD | 39 | 1 | 40 | 0 | VDD | GND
